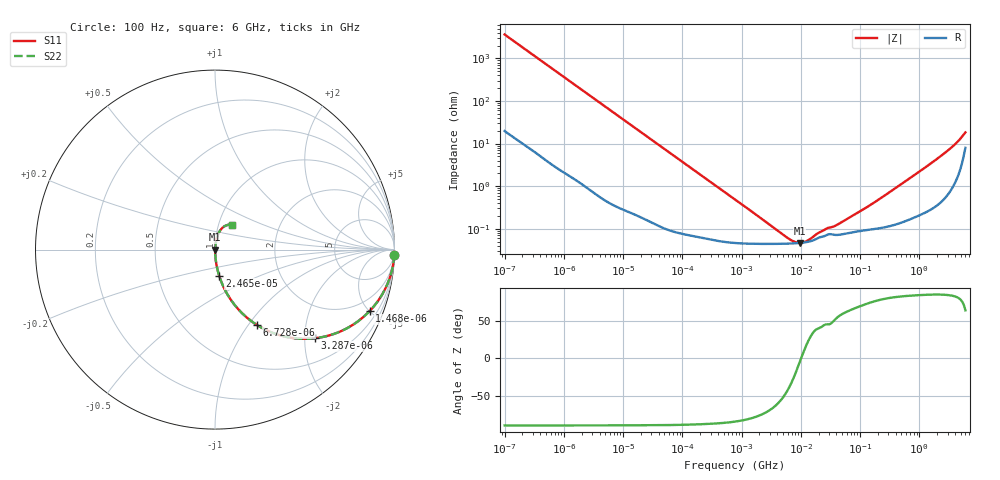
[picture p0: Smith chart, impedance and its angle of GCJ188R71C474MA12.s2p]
!Murata Part Number: GCJ188R71C474MA12
!These Parameters are Measured in Series Mode Connection
!Data Generated on Mar 13, 2026
!  o--ll--o
!Port1  Port2
!  o------o
!Operation Temp=25[degC], DC Bias Voltage=0[V]
!Freq. Start=100[Hz] Stop=6[GHz] 401[Steps]
# Hz S RI R 50
!Freq.(Hz) S11(Real) S11(Imag) S21(Real) S21(Imag) S12(Real) S12(Imag) S22(Real) S22(Imag)
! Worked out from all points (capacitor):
!   401 points, 100 Hz to 6 GHz, reference 50 ohm
!   read as one part in series: C = 436 nF near 109 Hz
!   lowest |Z| = 46.7 mohm at 9.506 MHz (marker M1)
!   series resonance near 10.11 MHz, so ESL is about 570 pH
!   S11 on the Smith chart (normalised r, x): 100 Hz: 1, -73; 1.468 kHz: 1.03, -5.01; 3.287 kHz: 1.01, -2.24; 6.728 kHz: 1.01, -1.10; 24.65 kHz: 1.00, -0.30; 6 GHz: 1.16, +0.33
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100  0.9991 -0.0274  0.000902 0.0274  0.000902 0.0274  0.9991 -0.0274
458  0.9839 -0.1231  0.0161 0.1231  0.0161 0.1231  0.9839 -0.1231
897  0.9425 -0.2301  0.0575 0.2301  0.0575 0.2301  0.9425 -0.2301
1468  0.861 -0.343  0.139 0.343  0.139 0.343  0.861 -0.343
2008  0.7692 -0.4183  0.2308 0.4183  0.2308 0.4183  0.7692 -0.4183
3287  0.5569 -0.4937  0.4431 0.4937  0.4431 0.4937  0.5569 -0.4937
6728  0.2332 -0.4196  0.7668 0.4196  0.7668 0.4196  0.2332 -0.4196
12041  0.0883 -0.2796  0.9117 0.2796  0.9117 0.2796  0.0883 -0.2796
24648  0.0237 -0.147  0.9763 0.147  0.9763 0.147  0.0237 -0.147
40335  0.00958 -0.0914  0.9904 0.0914  0.9904 0.0914  0.00958 -0.0914
129199  0.00154 -0.0289  0.9985 0.0289  0.9985 0.0289  0.00154 -0.0289
774597  0.000487 -0.00487  0.9995 0.00487  0.9995 0.00487  0.000487 -0.00487
5809218  0.000447 -0.000438  0.9996 0.000438  0.9996 0.000438  0.000447 -0.000438
9506416  0.000464 -4.6e-05  0.9995 4.6e-05  0.9995 4.6e-05  0.000464 -4.6e-05
1.189169e7  0.000482 0.000123  0.9995 -0.000123  0.9995 -0.000123  0.000482 0.000123
1.555665e7  0.000524 0.000336  0.9995 -0.000336  0.9995 -0.000336  0.000524 0.000336
2.035112e7  0.000623 0.000528  0.9994 -0.000528  0.9994 -0.000528  0.000623 0.000528
8.154455e7  0.000849 0.00199  0.9992 -0.00199  0.9992 -0.00199  0.000849 0.00199
3.124326e8  0.00119 0.00707  0.9988 -0.00707  0.9988 -0.00707  0.00119 0.00707
2.34314e9  0.00686 0.0511  0.9931 -0.0511  0.9931 -0.0511  0.00686 0.0511
4.385646e9  0.0266 0.1032  0.9734 -0.1032  0.9734 -0.1032  0.0266 0.1032
6e9  0.0947 0.1381  0.9053 -0.1381  0.9053 -0.1381  0.0947 0.1381
